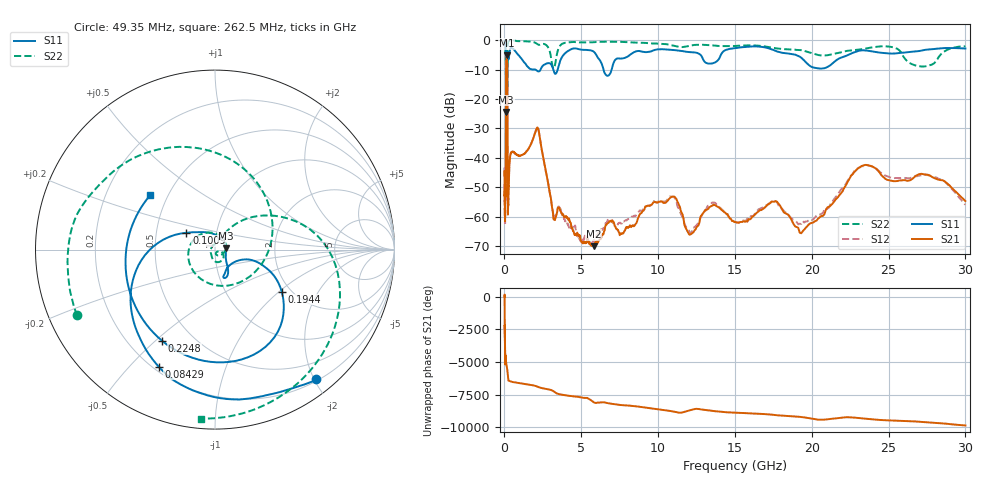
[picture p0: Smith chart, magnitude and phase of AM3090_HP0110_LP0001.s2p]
! Date/Time: Thu, Feb 28, 2019 1:59 PM
! Network Analyzer: Agilent Technologies E8364B Rev: A.07.50.67
! Sweep from 0.010 to 30.000 GHz, 1601 Points, Sweep Type: LOG
! Power Supply: 5.023 V, 0.002 A
# Hz S DB R 50
!freq MagS11 AngS11 MagS21 AngS21 MagS12 AngS12 MagS22 AngS22
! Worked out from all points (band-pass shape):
!   1601 points, 10 MHz to 30 GHz, reference 50 ohm
!   highest |S21| = -5.13 dB at 141.1 MHz (marker M1); lowest = -70.0 dB at 5.812 GHz (marker M2)
!   |S21| within 3 dB of the highest: 109 MHz to 178.9 MHz (69.85 MHz wide, 48.5 % of centre)
!   lowest |S11| = -24.4 dB at 107.7 MHz (marker M3), VSWR 1.13, Z = 56.3 + j1.01 ohm
!   |S11| at or under -10 dB: 2.002 GHz to 2.353 GHz (350.8 MHz wide, 16.1 % of centre); 3.18 GHz to 3.464 GHz (283.9 MHz wide, 8.55 % of centre); 6.447 GHz to 6.978 GHz (531.3 MHz wide, 7.92 % of centre)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
!   |S22| runs from -35.8 to -0.1 dB; largest |S21 - S12| = 0.012
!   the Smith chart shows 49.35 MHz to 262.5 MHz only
!   S11 on the Smith chart (normalised r, x): 49.35 MHz: 0.22, -2.03; 84.29 MHz: 0.22, -0.61; 100.9 MHz: 0.71, +0.14; 194.4 MHz: 1.80, -1.04; 224.8 MHz: 0.34, -0.52; 262.5 MHz: 0.40, +0.31
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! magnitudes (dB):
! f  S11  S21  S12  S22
! 10 MHz  -0.2  -45.9  -44.8  -0.5
! 38.04 MHz  -0.5  -59.1  -58.8  -1.3
! 49.35 MHz  -0.7  -51.3  -48.2  -1.4
! 84.29 MHz  -2.8  -48.9  -46.6  -6.0
! 100.9 MHz  -14.7  -14.6  -14.6  -15.3
! 107.7 MHz  -24.4  -8.7  -8.7  -18.7
! 141.1 MHz  -16.5  -5.1  -5.1  -32.6
! 144.7 MHz  -16.7  -5.1  -5.1  -27.2
! 171.5 MHz  -16.9  -6.7  -6.6  -32.9
! 194.4 MHz  -7.1  -20.6  -20.5  -8.9
! 224.8 MHz  -4.6  -59.0  -57.2  -1.2
! 262.5 MHz  -6.5  -52.6  -52.6  -0.5
! 550.5 MHz  -3.0  -37.9  -38.0  -0.2
! 2.084 GHz  -10.3  -30.1  -30.0  -1.2
! 3.22 GHz  -10.7  -60.9  -60.2  -9.6
! 5.812 GHz  -3.9  -70.0  -68.0  -0.7
! 7.926 GHz  -5.9  -63.5  -61.1  -0.7
! 10.81 GHz  -3.3  -53.4  -53.0  -1.7
! 12.19 GHz  -4.1  -65.7  -65.2  -1.8
! 19.61 GHz  -7.5  -63.7  -61.5  -3.8
! 23.59 GHz  -3.6  -42.4  -42.5  -2.8
! 30 GHz  -2.9  -54.6  -55.9  -2.2
